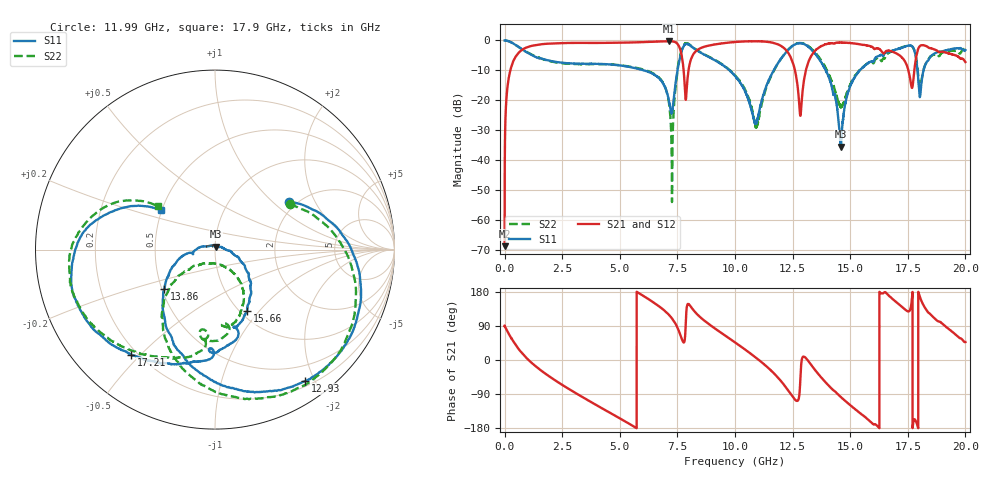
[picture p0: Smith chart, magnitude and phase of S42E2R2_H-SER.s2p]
! Created Wed Nov 25 21:39:43 2020
# khz S ma R 50
! 2 Port Network Data from SP1.SP block
! freq  magS11  angS11  magS21  angS21  magS12  angS12  magS22  angS22
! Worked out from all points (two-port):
!   20001 points, 300 kHz to 20 GHz, reference 50 ohm
!   highest |S21| = -0.24 dB at 7.12 GHz (marker M1); lowest = -68.8 dB at 300 kHz (marker M2)
!   |S21| within 3 dB of the highest: 737.5 MHz to 7.633 GHz (6.895 GHz wide, 165 % of centre); 8.357 GHz to 12.22 GHz (3.863 GHz wide, 37.5 % of centre)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
!   lowest |S11| = -35.5 dB at 14.59 GHz (marker M3), VSWR 1.03, Z = 50.5 + j1.62 ohm
!   |S11| at or under -10 dB: 6.048 GHz to 7.504 GHz (1.457 GHz wide, 21.5 % of centre); 9.765 GHz to 11.68 GHz (1.914 GHz wide, 17.9 % of centre); 13.94 GHz to 15.41 GHz (1.474 GHz wide, 10 % of centre)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
!   |S22| runs from -54.0 to 0.0 dB; largest |S21 - S12| = 0.021
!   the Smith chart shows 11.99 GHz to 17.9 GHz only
!   S11 on the Smith chart (normalised r, x): 11.99 GHz: 1.81, +1.28; 12.93 GHz: 0.27, -1.87; 13.86 GHz: 0.51, -0.26; 15.66 GHz: 1.07, -0.87; 17.21 GHz: 0.18, -0.47; 17.9 GHz: 0.50, +0.25
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300  0.9994 -0.2  0.0003645 89.8  0.0004035 90.8  0.9998 -0.2
126300  0.9844 -14.4  0.1687 75.3  0.1694 75.3  0.9848 -14.4
451300  0.8537 -47.8  0.5146 42.4  0.516 42.5  0.8547 -47.9
1482300  0.5055 -113.5  0.8501 -22.9  0.8509 -23.0  0.519 -113.1
3334300  0.4083 171.3  0.9108 -96.2  0.9104 -96.2  0.4027 175.8
6667300  0.2402 64.0  0.9588 143.3  0.9576 143.2  0.2454 47.1
7120300  0.1041 61.1  0.9725 119.9  0.9703 119.9  0.09849 23.4
7280300  0.06677 127.7  0.9644 108.5  0.9643 108.5  0.01242 -177.1
7881300  0.8746 92.3  0.1148 121.3  0.1135 121.2  0.9009 83.2
1.00003e7  0.2555 -40.4  0.9419 46.5  0.9428 46.6  0.2622 -49.1
1.09363e7  0.04313 21.6  0.9695 4.9  0.9692 4.9  0.03559 175.5
1.19873e7  0.4898 33.1  0.8156 -55.0  0.8178 -54.8  0.4876 31.3
1.29333e7  0.8878 -55.5  0.1415 7.0  0.143 6.9  0.8934 -62.8
1.33343e7  0.6937 -96.9  0.5711 -15.2  0.5714 -15.7  0.7148 -101.3
1.38603e7  0.3592 -142.1  0.8397 -54.1  0.8333 -54.2  0.3945 -135.8
1.45923e7  0.01675 73.2  0.9236 -97.4  0.9256 -97.3  0.07684 -99.6
1.56603e7  0.3872 -62.6  0.8336 -151.3  0.8433 -151.3  0.3882 -69.0
1.66673e7  0.6399 -101.8  0.6759 170.7  0.6608 170.4  0.6223 -105.1
1.72073e7  0.7492 -128.4  0.5356 142.5  0.5241 142.7  0.7563 -136.2
1.79043e7  0.3718 144.0  0.6328 -170.2  0.6334 -170.3  0.3965 142.9
1.84483e7  0.5157 -139.1  0.7456 122.7  0.7445 123.0  0.5233 -153.4
2e7  0.6909 154.7  0.4362 47.4  0.4381 48.4  0.7545 143.6
